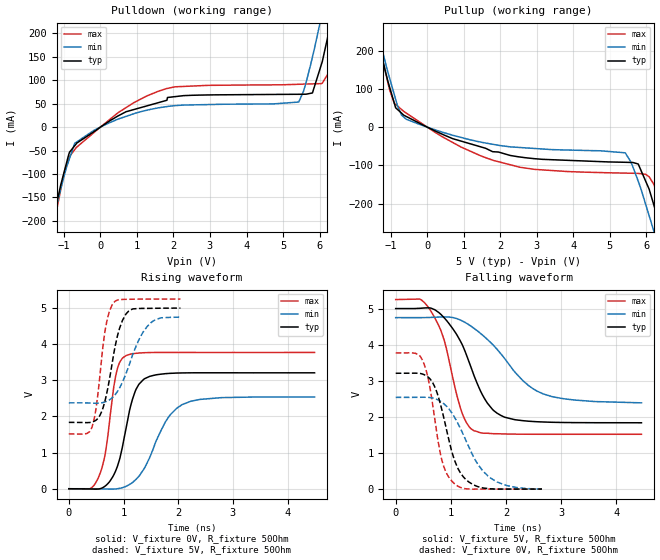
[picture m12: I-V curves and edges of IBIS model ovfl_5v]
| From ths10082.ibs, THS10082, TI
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|   ovfl_5v Model
[Model]   ovfl_5v
Model_type   Output
Polarity   Non-Inverting
Vmeas = 2.5
Vref = 2.5
Cref = 2pF
Rref = 50
|   typ   min   max
C_comp   1.852e-12   1.842e-12   1.893e-12
[Voltage Range]   5   4.75   5.25
|Ambient Temperature   25   85   -40
|Junction Temperature
[Temperature Range]   27   125   -40
[Pullup Reference]   5   4.75   5.25
[Pulldown Reference]   0   0   0
[Power Clamp Reference]   5   4.75   5.25
[GND Clamp Reference]   0   0   0
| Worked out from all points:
|   slope of the pulldown table from 0 to 0.75 V, typ, clamps not added: 22.1 ohm
|   slope of the pullup table from 0 to 0.75 V, typ, clamps not added: 23.8 ohm
|   falling waveform, V_fixture 5V, R_fixture 50Ohm: 20-80 % time 557ps typ, 851ps min, 382ps max; typ from 5 V to 1.84 V
|   rising waveform, V_fixture 0V, R_fixture 50Ohm: 20-80 % time 291ps typ, 492ps min, 208ps max; typ from 0 V to 3.21 V
|   rising waveform, V_fixture 5V, R_fixture 50Ohm: 20-80 % time 246ps typ, 387ps min, 177ps max; typ from 1.84 V to 5 V
|   falling waveform, V_fixture 0V, R_fixture 50Ohm: 20-80 % time 337ps typ, 527ps min, 251ps max; typ from 3.21 V to 0 V
[Pulldown]
|   Voltage   I(typ)   I(min)   I(max)
-5V       -1.695A    -1.561A    -1.837A
-1.302V   -199.7mA   -200.1mA   -217.6mA
-997.5mV  -97.5mA    -105.9mA   -99.34mA
-703mV    -39.75mA   -34.59mA   -48.12mA
924mV     37.72mA    28.84mA    52.67mA
2.042V    65.11mA    45.92mA    86.09mA
5.425V    70.14mA    53.56mA    91.49mA
5.805V    73.01mA    149.7mA    92.39mA
6.053V    134.7mA    236.9mA    92.97mA
6.3V      219.4mA    324.9mA    134.9mA
6.525V    302.9mA    405.2mA    217.5mA
10V       1.73A      1.786A     1.677A
[Pullup]
|   Voltage   I(typ)   I(min)   I(max)
-5V       1.777A     1.721A     1.836A
-2.622V   754.9mA    746.6mA    788.5mA
-1.31V    209.7mA    229.6mA    210.6mA
-903mV    62.94mA    85.39mA    62.4mA
-703mV    36.52mA    31.29mA    46.11mA
251.7mV   -11.6mA    -8.176mA   -15.71mA
2.541V    -78.04mA   -53.2mA    -104.9mA
5.415V    -91.78mA   -67.01mA   -120.1mA
5.775V    -96.33mA   -141.3mA   -120.7mA
6.205V    -204.2mA   -272.5mA   -149.8mA
6.557V    -324.3mA   -382.3mA   -271.2mA
10V       -1.698A    -1.653A    -1.741A
[Ramp]
R_load = 50
|   typ   min   max
dV/dt_r   1.92515/2.89299e-10   1.52416/4.89712e-10   2.26293/2.07067e-10
dV/dt_f   1.89784/5.56605e-10   1.42308/8.56903e-10   2.23898/3.82155e-10
[Falling Waveform]
V_fixture = 5V
V_fixture_min = 4.75V
V_fixture_max = 5.25V
R_fixture = 50Ohm
|   Time   V(typ)   V(min)   V(max)
0s        5V         4.75V      5.25V
436ps     5.007V     4.749V     5.263V
644ps     5.01V      4.756V     4.917V
882ps     4.742V     4.769V     4.118V
1.202ns   4.018V     4.663V     2.122V
1.416ns   3.167V     4.459V     1.619V
1.842ns   2.1V       3.869V     1.533V
2.306ns   1.896V     3.008V     1.52V
2.674ns   1.859V     2.638V     1.518V
4.46ns    1.837V     2.389V     1.519V
[Rising Waveform]
V_fixture = 0V
V_fixture_min = 0V
V_fixture_max = 0V
R_fixture = 50Ohm
|   Time   V(typ)   V(min)   V(max)
0s        1.848nV    2.664nV    1.618nV
544ps     -7.17mV    -2.487mV   320.9mV
670ps     80.38mV    -6.507mV   1.013V
854ps     486.4mV    -5.771mV   3.103V
1.046ns   1.671V     66.52mV    3.685V
1.216ns   2.708V     241.4mV    3.746V
1.368ns   3.027V     535mV      3.764V
1.762ns   3.185V     1.843V     3.773V
2.072ns   3.205V     2.329V     3.772V
4.492ns   3.209V     2.54V      3.772V
[Rising Waveform]
V_fixture = 5V
V_fixture_min = 4.75V
V_fixture_max = 5.25V
R_fixture = 50Ohm
|   Time   V(typ)   V(min)   V(max)
0s        1.837V     2.378V     1.518V
424ps     1.846V     2.37V      1.708V
514ps     1.92V      2.367V     2.403V
672ps     2.499V     2.409V     4.453V
822ps     3.745V     2.561V     5.152V
930ps     4.45V      2.797V     5.237V
1.092ns   4.913V     3.376V     5.243V
1.288ns   4.99V      4.145V     5.248V
1.508ns   4.993V     4.607V     5.25V
2.04ns    5V         4.749V     5.25V
[Falling Waveform]
V_fixture = 0V
V_fixture_min = 0V
V_fixture_max = 0V
R_fixture = 50Ohm
|   Time   V(typ)   V(min)   V(max)
0s        3.209V     2.54V      3.772V
486ps     3.187V     2.544V     3.57V
604ps     3.082V     2.538V     2.954V
736ps     2.73V      2.492V     1.663V
840ps     2.184V     2.404V     792.2mV
1.054ns   861.3mV    2.024V     166.2mV
1.27ns    269mV      1.362V     9.118mV
1.496ns   65.72mV    675.7mV    246.7uV
1.694ns   9.852mV    334.4mV    363uV
2.654ns   463.3uV    2.547mV    173.6uV
